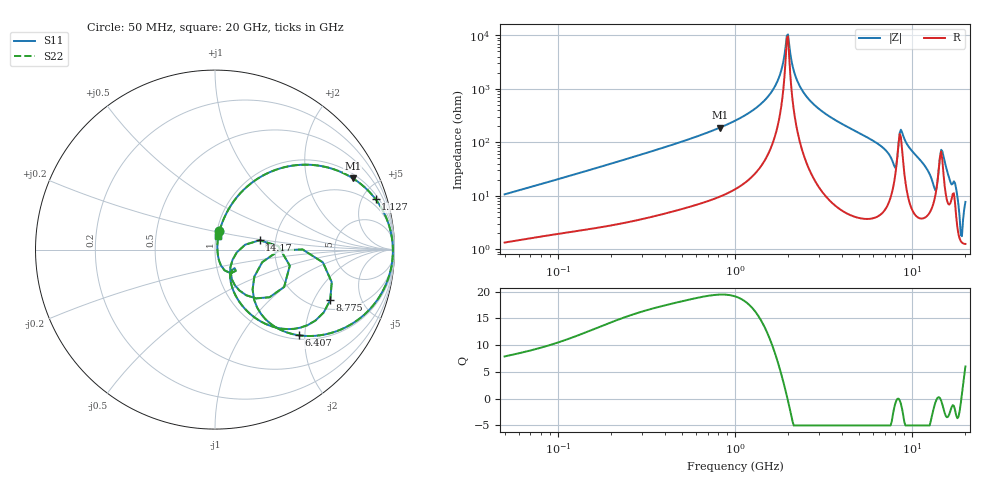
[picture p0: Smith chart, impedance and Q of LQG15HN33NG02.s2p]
!Murata Part Number: LQG15HN33NG02
!These Parameters are Measured in Series Mode Connection
!  o--[Z]--o
!Port1  Port2
!  o-------o
!Freq. Start=50[MHz] Stop=20[GHz], 401[Steps]
# Hz S RI R 50
!Freq.(Hz) S11(Real) S11(Imag) S21(Real) S21(Imag) S12(Real) S12(Imag) S22(Real) S22(Imag)
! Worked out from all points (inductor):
!   401 points, 50 MHz to 20 GHz, reference 50 ohm
!   read as one part in series: L = 32.9 nH near 51.52 MHz
!   highest Q = 19.4 at 823.1 MHz (marker M1), where L = 36.3 nH
!   self-resonance near 1.962 GHz
!   S11 on the Smith chart (normalised r, x): 50 MHz: 1.03, +0.21; 1.127 GHz: 1.34, +6.23; 6.407 GHz: 1.08, -1.87; 8.775 GHz: 2.46, -2.71; 14.17 GHz: 1.65, +0.18; 20 GHz: 1.03, +0.15
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5e7  0.0237 0.1013  0.9763 -0.1013  0.9763 -0.1013  0.0237 0.1013
1.364002e8  0.0873 0.2439  0.9127 -0.2439  0.9127 -0.2439  0.0873 0.2439
3.721004e8  0.3654 0.4533  0.6346 -0.4533  0.6346 -0.4533  0.3654 0.4533
8.230629e8  0.7677 0.3974  0.2323 -0.3974  0.2323 -0.3974  0.7677 0.3974
1e9  0.8513 0.3306  0.1487 -0.3306  0.1487 -0.3306  0.8513 0.3306
1.127304e9  0.8943 0.2813  0.1057 -0.2813  0.1057 -0.2813  0.8943 0.2813
1.639343e9  0.9791 0.1002  0.0209 -0.1002  0.0209 -0.1002  0.9791 0.1002
1.99176e9  0.9911 -0.00354  0.00891 0.00354  0.00891 0.00354  0.9911 -0.00354
2.245319e9  0.987 -0.0687  0.013 0.0687  0.013 0.0687  0.987 -0.0687
2.728004e9  0.9603 -0.1748  0.0397 0.1748  0.0397 0.1748  0.9603 -0.1748
6.406762e9  0.4679 -0.4775  0.5321 0.4775  0.5321 0.4775  0.4679 -0.4775
7.442007e9  0.2777 -0.3841  0.7223 0.3841  0.7223 0.3841  0.2777 -0.3841
8.020766e9  0.2192 -0.1504  0.7808 0.1504  0.7808 0.1504  0.2192 -0.1504
8.389408e9  0.4877 0.000842  0.5123 -0.000842  0.5123 -0.000842  0.4877 0.000842
8.774992e9  0.6421 -0.2808  0.3579 0.2808  0.3579 0.2808  0.6421 -0.2808
9.892087e9  0.3488 -0.4365  0.6512 0.4365  0.6512 0.4365  0.3488 -0.4365
1.334722e10  0.0863 -0.097  0.9137 0.097  0.9137 0.097  0.0863 -0.097
1.417136e10  0.2487 0.052  0.7513 -0.052  0.7513 -0.052  0.2487 0.052
1.504638e10  0.3041 -0.2654  0.6959 0.2654  0.6959 0.2654  0.3041 -0.2654
1.747767e10  0.0877 -0.1317  0.9123 0.1317  0.9123 0.1317  0.0877 -0.1317
1.88369e10  0.0141 -0.0115  0.9859 0.0115  0.9859 0.0115  0.0141 -0.0115
2e10  0.0179 0.0733  0.9821 -0.0733  0.9821 -0.0733  0.0179 0.0733
